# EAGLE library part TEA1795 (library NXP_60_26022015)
The TEA1795T is a member of the new generation of Synchronous Rectifier (SR) controller ICs for switched mode power supplies. Its high level of integration enables the design of a cost-effective power supply with a minimum number of external components. AAL Eindhoven MK
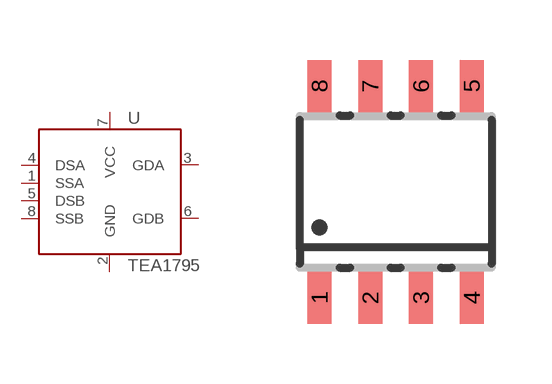
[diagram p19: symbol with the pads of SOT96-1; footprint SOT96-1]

Designator prefix U

## TEA1795T (12NC: 9352 915 64118)  [SOT96-1]
1  SSA  in
2  GND  pwr
3  GDA  out
4  DSA  in
5  DSB  in
6  GDB  out
7  VCC  pwr
8  SSB  in

## Footprint SOT96-1 (pad centres in mm)
SOT96-1 SO8: plastic small outline package; 8 leads; body width 3.9 mm JEDEC: MS-012 IEC: 076E03
smd 0.6 x 1.3: 1 -1.905,-2.65; 2 -0.635,-2.65; 3 0.635,-2.65; 4 1.905,-2.65; 5 1.905,2.65; 6 0.635,2.65; 7 -0.635,2.65; 8 -1.905,2.65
